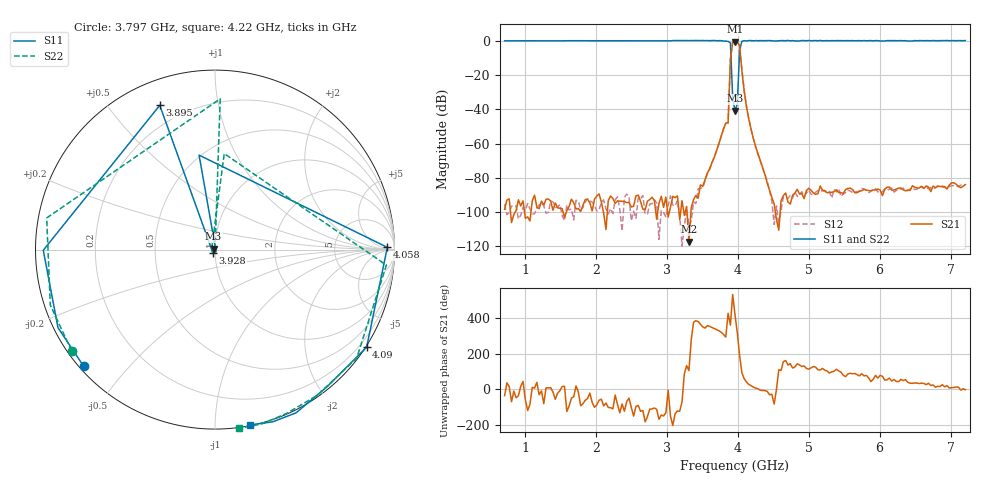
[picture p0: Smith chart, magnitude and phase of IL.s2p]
!Agilent Technologies,E8364B,MY43040703,A.07.50.48
!Agilent E8364B: A.07.50.48
!Date: Wednesday, April 10, 2024 15:25:51
!Correction: S11(Full 2 Port(1,2))
!S21(Full 2 Port(1,2))
!S12(Full 2 Port(1,2))
!S22(Full 2 Port(1,2))
!S2P File: Measurements: S11, S21, S12, S22:
# Hz S  dB  R 50
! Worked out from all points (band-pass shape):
!   201 points, 710 MHz to 7.21 GHz, reference 50 ohm
!   highest |S21| = -0.59 dB at 3.96 GHz (marker M1); lowest = -117.2 dB at 3.31 GHz (marker M2)
!   |S21| within 3 dB of the highest: 3.919 GHz to 4.027 GHz (108 MHz wide, 2.72 % of centre)
!   lowest |S11| = -40.7 dB at 3.96 GHz (marker M3), VSWR 1.02, Z = 49.2 + j0.422 ohm
!   |S11| at or under -10 dB: 3.904 GHz to 4.02 GHz (116.5 MHz wide, 2.94 % of centre)
!   |S22| runs from -34.4 to 0.2 dB; largest |S21 - S12| = 0.011
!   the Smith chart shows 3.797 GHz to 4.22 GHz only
!   S11 on the Smith chart (normalised r, x): 3.797 GHz: 0.01, -0.38; 3.895 GHz: 0.11, +0.68; 3.928 GHz: 0.98, -0.03; 4.058 GHz: 45, +14; 4.09 GHz: -0.03, -3.40; 4.22 GHz: 0.00, -1.22
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7.1e8  -0.06 121.9  -98.31 -36.5  -95.39 81.8  -0.10 119.3
1.2625e9  -0.01 78.7  -95.84 -81.1  -96.17 -23.2  -0.07 75.0
1.815e9  0.04 37.3  -96.04 -82.0  -97.30 -69.2  -0.01 33.0
2.3025e9  -0.01 2.4  -93.53 -85.0  -91.07 -80.9  0.02 -1.9
2.8875e9  0.00 -38.8  -94.85 -169.2  -115.88 -145.2  -0.04 -43.1
3.31e9  0.10 -70.0  -117.18 104.1  -108.01 111.9  -0.00 -74.1
3.5375e9  0.07 -90.9  -80.98 -17.2  -81.72 -12.4  0.11 -94.7
3.7e9  0.04 -112.3  -64.08 -25.9  -64.17 -26.2  0.10 -117.5
3.7975e9  -0.19 -138.3  -51.47 -52.6  -51.51 -52.6  -0.19 -144.7
3.8625e9  -0.38 -179.8  -47.92 65.7  -47.87 65.8  -0.41 169.4
3.895e9  -1.30 110.9  -10.94 -0.4  -10.86 -0.2  -1.51 88.0
3.9275e9  -33.45 -123.6  -0.81 171.0  -0.72 170.7  -33.78 -91.1
3.96e9  -40.74 152.1  -0.59 57.4  -0.51 57.3  -33.03 -127.4
3.9925e9  -37.06 -64.2  -0.59 -44.2  -0.55 -44.1  -34.36 177.6
4.025e9  -5.45 99.6  -2.90 -171.5  -2.80 -171.8  -5.39 84.5
4.0575e9  -0.35 0.7  -17.40 91.3  -17.28 91.4  -0.37 -5.2
4.09e9  0.04 -32.7  -29.34 58.0  -29.29 57.9  -0.05 -37.4
4.22e9  -0.03 -78.6  -57.30 11.5  -57.34 10.9  0.05 -82.2
4.415e9  0.08 -104.4  -83.12 -12.2  -81.86 -18.6  0.05 -107.5
5.065e9  0.07 -151.8  -88.79 126.9  -90.03 111.4  0.05 -154.4
6.1375e9  0.05 148.6  -85.35 62.4  -86.58 62.3  0.02 144.2
7.21e9  0.13 92.3  -83.92 -2.9  -84.00 -1.2  0.16 88.2
